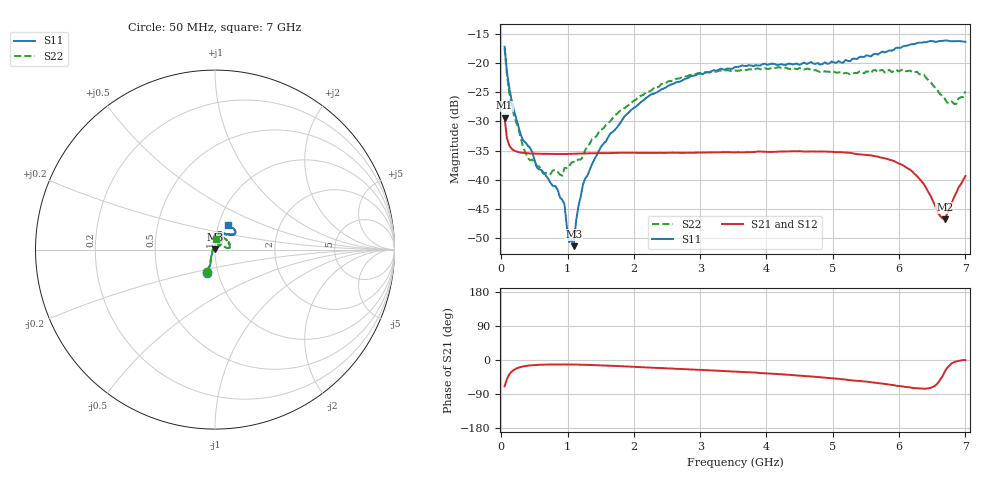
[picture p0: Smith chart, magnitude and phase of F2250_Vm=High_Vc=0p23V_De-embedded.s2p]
! Integrated Device Technology
! Corporate Headquarters
! 6024 Silver Creek Valley Road
! San Jose, CA 95138  USA
! Phone:  1-408-284-8200
! Toll Free:  1-800-223-1366
! Webpage:  http://www.idt.com/
! Timing and RF Division
! 515 Groton Road, Suite 102
! Westford, MA 01886-6024
! Device:  F2250
! Description: Voltage Variable RF Attenuator
! Frequency:  50.0 -  6000.00 MHz
! Package:  3x3 mm Thin QFN Plastic Package: 16 pin
! Ports:  2 RF, 3 DC
!  Pin  1  = GND
!  Pin  2  = NC
!  Pin  3  = RF1  = Port 1
!  Pin  4  = NC
!  Pin  5  = GND
!  Pin  6  = GND
!  Pin  7  = GND
!  Pin  8  = GND
!  Pin  9  = NC
!  Pin 10  = RF2  = Port 2
!  Pin 11  = NC
!  Pin 12  = GND
!  Pin 13  = GND
!  Pin 14  = VCNTRL
!  Pin 15  = VDD
!  Pin 16  = VMODE
! Vcntrl:  0.230 Volts
! Vmode:  +3.300 Volts
! Vdd:  +3.30  Volts
! Current:  1.247 mA
! Data:  The device was measured on a the F2250 evaluation board which has
!  individual transmission lines to the RF pins.  Data was collected
!  using a calibrated network analyzer.  The evaluation board was
!  de-embedded using a TRL calibration technique.
!  The reference plane is the edge of the package pin.
! Misc:  SN 10
!  Action Tracker AT0258
! Date Measured:  2014-11-26
! Date:  2015-10-15  MJV
! Note:
!  Integrated Device Technology supplies this data as a sample of measured
!  data at the package pin for this product.  Your particular data for this
!  product may vary.
!  Data was taken at 25 degrees C.
!  Integrated Device Technology reserves the right to change this data at anytime.
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# GHz S dB R 50
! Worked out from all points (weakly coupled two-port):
!   201 points, 50 MHz to 7 GHz, reference 50 ohm
!   highest |S21| = -29.38 dB at 50 MHz (marker M1); lowest = -46.8 dB at 6.687 GHz (marker M2)
!   lowest |S11| = -51.4 dB at 1.093 GHz (marker M3), VSWR 1.01, Z = 50 + j0.269 ohm
!   |S11| at or under -10 dB: start of sweep to end of sweep
!   |S22| runs from -39.3 to -17.4 dB; largest |S21 - S12| = 6.3e-05
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0.05  -17.18 -108.5  -29.38 -69.5  -29.38 -69.5  -17.38 -110.5
0.08475  -21.47 -107.4  -32.85 -50.1  -32.85 -50.0  -21.89 -108.9
0.15425  -26.23 -116.6  -34.67 -31.0  -34.67 -31.0  -27.14 -120.4
0.29325  -32.27 -127.4  -35.34 -18.4  -35.34 -18.4  -32.74 -133.3
0.3975  -34.11 -142.1  -35.47 -15.0  -35.47 -15.1  -36.21 -158.3
0.5365  -37.90 -154.7  -35.54 -12.9  -35.54 -13.0  -37.63 -179.6
0.64075  -38.77 -162.5  -35.57 -12.2  -35.57 -12.2  -39.06 160.5
0.91875  -43.45 156.1  -35.59 -11.8  -35.59 -11.8  -39.33 127.2
0.9535  -44.22 170.7  -35.59 -11.8  -35.59 -11.8  -37.97 123.7
1.023  -50.73 140.2  -35.58 -11.9  -35.58 -11.9  -37.78 107.2
1.0925  -51.42 89.9  -35.56 -12.0  -35.56 -12.0  -36.92 97.7
1.12725  -47.15 61.6  -35.55 -12.1  -35.56 -12.1  -36.93 91.1
1.2315  -40.85 40.7  -35.52 -12.5  -35.52 -12.5  -36.08 76.5
1.6485  -32.03 41.2  -35.43 -15.2  -35.43 -15.2  -29.92 59.6
2.37825  -24.76 46.7  -35.39 -21.1  -35.39 -21.0  -24.03 53.8
3.525  -20.65 71.7  -35.31 -30.6  -35.31 -30.7  -21.27 72.9
4.7065  -20.06 72.0  -35.14 -43.9  -35.15 -43.9  -21.23 70.3
5.85325  -17.79 40.5  -36.58 -64.9  -36.57 -65.0  -21.14 23.3
6.27025  -16.53 39.4  -39.38 -74.5  -39.40 -74.6  -21.47 8.5
6.68725  -16.11 47.9  -46.78 -31.2  -46.77 -31.0  -26.05 28.3
6.861  -16.22 54.5  -42.31 -3.8  -42.28 -3.8  -27.00 57.4
7  -16.32 62.4  -39.36 -0.2  -39.33 -0.4  -24.83 83.7
